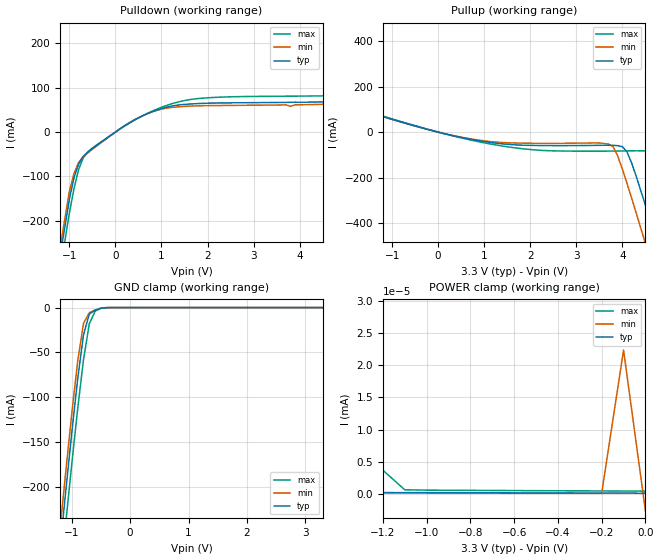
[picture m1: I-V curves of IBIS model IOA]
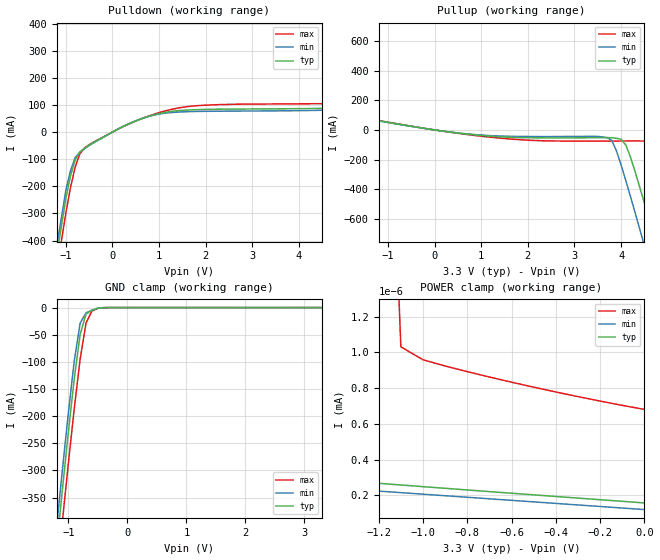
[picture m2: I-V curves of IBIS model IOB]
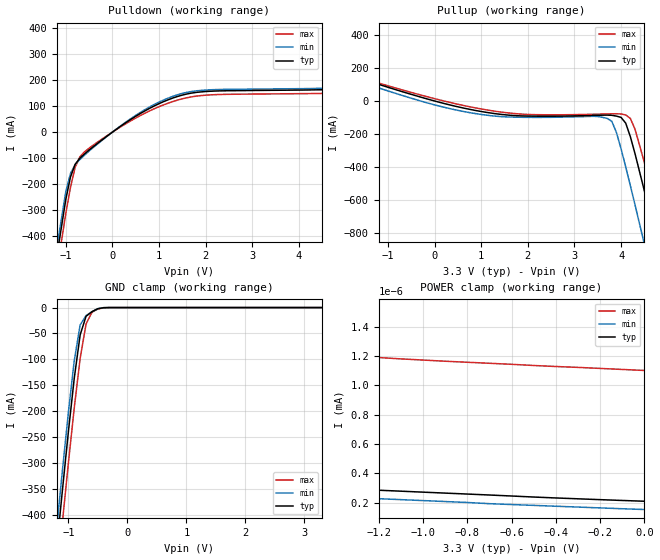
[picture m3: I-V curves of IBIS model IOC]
| IBIS file Qspan.ibs created by s2ibis2 version 2.1
[IBIS ver]   2.1
[File name]   qspn25a.ibs
[File Rev]   1.1
[Date]   10-17-2000
[Notes]   The data is simulation based
|   History : #3591862.MI003.01 - Original Model
|   #3591862.MI003.02 - Revised Power Pins.
|   #3591862.MI003.03 - Fixed IOA, IOB, and IOE Clamp
|   Characteristics and removed INE.
|   #3591862.MI003.04 - Updated with IDT formatting.
|   This is the Qspan II (CA91L862A-XXL, 17mm PBGA) IBIS
|   MODEL for a 5 V PCI signalling environment.
[Disclaimer] This model is subject to change.
   Integrated Device Technology, Inc. ("IDT") hereby grants the
   user of this IBIS model a non-exclusive, nontransferable
   license to use this IBIS model under the following terms. The
   user is granted this license only to use the IBIS model and is
   not granted rights to sell, copy (except as needed to run the
   IBIS model), rent, lease or sub-license the IBIS model in
   whole or in part, or in modified form to anyone. The User may
   modify the IBIS model to suit its specific applications, but
   rights to derivative works and such modifications shall belong
   to IDT. This IBIS model is provided on an AS IS" basis and IDT
   makes absolutely no warranty with respect to the information
   contained herein. IDT DISCLAIMS AND CUSTOMER WAIVES ALL
   WARRANTIES, EXPRESS AND IMPLIED, INCLUDING WARRANTIES OF
   MERCHANTABILITY AND FITNESS FOR A PARTICULAR PURPOSE. THE
   ENTIRE RISK AS TO QUALITY AND PERFORMANCE IS WITH THE USER
   ACCORDINGLY, IN NO EVENT SHALL IDT BE LIABLE FOR ANY DIRECT OR
   INDIRECT DAMAGES, WHETHER IN CONTRACT OR TORT, INCLUDING ANY
   LOST PROFITS OR OTHER INCIDENTAL, CONSEQUENTIAL, EXEMPLARY, OR
   PUNITIVE DAMAGES ARISING OUT OF THE USE OR APPLICATION OF THE
   IBIS model. Further, IDT reserves the right to make changes
   without notice to any product herein to improve reliability,
   function, or design. IDT does not convey any license under
   patent rights or any other intellectual property rights,
   including those of third parties. IDT is not obligated to
   provide maintenance or support for the licensed IBIS model.
[Copyright]   Copyright 2009, Integrated Device Technology, Inc. all
   rights reserved.
|   Component QSPAN
[Component]   QSPAN
[Manufacturer]   Integrated Device Technology, Inc.
[Package]
| variable   typ   min   max
R_pkg   45m   22m   75m
L_pkg   2.5nH   1.1nH   4.3nH
C_pkg   1.3pF   1.2pF   1.4pF
[Pin]  signal_name   model_name
B3	D26		IOA
C3	D27		IOA
B1	D28		IOA
D3	D29		IOA
D2	D30		IOA
C2	D31		IOA
C1	A26		IOA
E3	A27		IOA
E4	A28		IOA
E1	A29		IOA
F3	A30		IOA
F2	A31		IOA
D1	R/W		IOA
F1	DSACK1/TA	IOB
G3	DSACK0   IOB
F4	SIZ1		IOA
G2	SIZ0		IOA
G1	SDA		IOB
H3	SCL		OUTA
H4	IMSEL		INA
K8	VSS		GND
H1	TMODE1	IOD
J3	TMODE0	IOD
J4	RESETI	INB
K1	RESETO	IOF
L4	BURST/TIP	IOA
K2	TS		IOB
L2	BB/BGACK	IOB
L1	BR		OUTA
M4   REQ   IOC
N2	AD31		IOC
P1	AD30		IOC
P2	AD29		IOC
N4	AD28		IOC
N3	AD27		IOC
M1	HALT/RETRY IOB
M3	GNT		IOC
M2	RST		INC
P8	PCLK		INC
J14	BM_EN		IOD
P3	AD26		IOC
R3	AD25		IOC
R2	AD24		IOC
T2	C/BE3		IOC
T1	AD23		IOC
N5	AD22		IOC
P5	AD21		IOC
N6	AD20		IOC
R6	AD19		IOC
T5	AD18		IOC
T6	AD17		IOC
P6	AD16		IOC
N7	C/BE2		IOC
P7	FRAME		IOC
R7	IRDY		IOC
N8	TRDY		IOC
R8	DEVSEL	IOC
T7	STOP		IOC
N9	PERR		IOC
N10	PAR		IOC
R9	C/BE1		IOC
P9	AD15		IOC
T8	AD14		IOC
T9	AD13		IOC
R10	AD12		IOC
P10	AD11		IOC
N11	AD10		IOC
P11	AD9		IOC
T10	AD8		IOC
R11	C/BE0		IOC
N12	IDSEL		INC
P12	AD7		IOC
P14	AD6		IOC
T13	AD5		IOC
T14	AD4		IOC
P15	AD3		IOC
T16	AD2		IOC
N14	AD1		IOC
N15	AD0		IOC
M13	CSREG		INA
P16	CSPCI		INA
N16	TC0		IOA
L14	TC1		IOA
M16	TC2		IOA
L13	TC3		IOA
L15	BERR/TEA	IOB
L16	AS		IOB
K14	BDIP		IOA
K16	BG		INA
H15	ENID		IOD
J13	DACK/SDACK	INB
J15	DONE		INA
H16	QINT		IOE
G13	DREQ		OUTA
M14	INT		IOC
M15	SERR		IOC
G14	A0		IOA
G16	A1		IOA
G15	A2		IOA
F14	A3		IOA
F16	A4		IOA
E16	A5		IOA
F15	D0		IOA
E15	D1		IOA
E14	D2		IOA
D16	D3		IOA
D15	D4		IOA
F13	D5		IOA
F6	VSS		GND
D8	QCLK		INA
F7	VSS		GND
F8	VSS		GND
E13	D6		IOA
D14	D7		IOA
C16	D8		IOA
C15	D9		IOA
B14	D10		IOA
B15	D11		IOA
C13	A6		IOA
B16	A7		IOA
C14	A8		IOA
A15	A9		IOA
D12	A10		IOA
C11	A11		IOA
D11	A12		IOA
A13	A13		IOA
A12	A14		IOA
B11	A15		IOA
C10	DS		OUTA
D10	D12		IOA
A11	D13		IOA
D9	D14		IOA
B10	D15		IOA
C9	D16		IOA
A10	D17		IOA
B9	D18		IOA
C8	D19		IOA
A9	A16		IOA
D7	A17		IOA
B8	A18		IOA
C7	A19		IOA
A8	A20		IOA
A7	A21		IOA
B7	A22		IOA
D6	A23		IOA
C6	A24		IOA
A6	A25		IOA
B6	D20		IOA
D5	D21		IOA
A4	D22		IOA
A3	D23		IOA
B4	D24		IOA
A2	D25		IOA
H13  TCK   INF
K15  TDI   INF
K13  TDO   OUTA
J16  TMS   INF
H14  TRST   INF
G4   ENUM   IOF
K4   HS_HEALTHY IOD
H2   HS_LED   IOF
J2   HS_SWITCH  IOD
K3   PCI_DIS   IOD
J1   PME   IOF
D4   DP3   IOA
B5   DP2   IOA
C5   DP1   IOA
A5   DP0   IOA
C4   PCI_ARB_EN  IOD
B12  BIDIR_CTRL/Test1 ING
A14  RAM_WE/Test2 IOD
C12  TMODE[2]/Test3 IOD
R1	EXT_GNT[1]  OUTB
R4	EXT_GNT[2]  OUTB
T3	EXT_GNT[3]  OUTB
P4	EXT_GNT[4]  OUTB
R5	EXT_GNT[5]  OUTB
T4	EXT_GNT[6]  OUTB
T11	EXT_REQ[1]  IOC
R12	EXT_REQ[2]  IOC
N13	EXT_REQ[3]  IOC
P13	EXT_REQ[4]  IOC
T12	EXT_REQ[5]  IOC
R13	EXT_REQ[6]	  IOC
N1   VH   POWER
R15   VH   POWER
B2   VH   POWER
A16   VH   POWER
F9   VSS   GND
F10   VSS   GND
E5   VDD   POWER
F11   VSS   GND
E6   VDD   POWER
G6   VSS   GND
E7   VDD   POWER
G7   VSS   GND
G8   VSS   GND
E8   VDD   POWER
E9   VDD   POWER
E10   VDD   POWER
G9   VSS   GND
G10   VSS   GND
E11   VDD   POWER
E12   VDD   POWER
G11   VSS   GND
F5   VDD   POWER
F12   VDD   POWER
H6   VSS   GND
G5   VDD   POWER
G12   VDD   POWER
H5   VDD   POWER
H12   VDD   POWER
J5   VDD   POWER
J12   VDD   POWER
K5   VDD   POWER
K12   VDD   POWER
L5   VDD   POWER
L12   VDD   POWER
M5   VDD   POWER
M6   VDD   POWER
M7   VDD   POWER
M8   VDD   POWER
M9   VDD   POWER
M10   VDD   POWER
M11   VDD   POWER
M12   VDD   POWER
H7   VSS   GND
H8   VSS   GND
H9   VSS   GND
H10   VSS   GND
H11   VSS   GND
J6   VSS   GND
J7   VSS   GND
J8   VSS   GND
J9   VSS   GND
J10   VSS   GND
J11   VSS   GND
K6   VSS   GND
K7   VSS   GND
K9   VSS   GND
K10   VSS   GND
K11   VSS   GND
L6   VSS   GND
L7   VSS   GND
L8   VSS   GND
L9   VSS   GND
L10   VSS   GND
L11   VSS   GND
| Models and submodels in the file (14): IOA (I/O), IOB (I/O), IOC (I/O), IOD (I/O), IOE (I/O), IOF (I/O), INA (Input), INB (Input), INC (Input), IND (Input), INF (Input), ING (Input), OUTA (Output), OUTB (Output)
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|   Model IOA
[Model]   IOA
Model_type   I/O
Polarity   Non-Inverting
Vinl =   0.8000V
Vinh =   2.0000V
C_comp   5.00pF   5.00pF   5.00pF
[Voltage Range]   3.3000V   3.0000V   4.0000V
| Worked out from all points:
|   slope of the pulldown table from 0 to 0.495 V, typ, clamps not added: 15.7 ohm
|   slope of the pullup table from 0 to 0.495 V, typ, clamps not added: 21.3 ohm
|   GND clamp passes 1 mA (typ) near -0.51 V on its own axis
|   POWER clamp passes 1 mA (typ) near -2.40 V on its own axis
[Pulldown]
| voltage   I(typ)   I(min)   I(max)
-3.3V     -1.71A     -1.69A     -1.742A
-1.5V     -470.3mA   -448.8mA   -505mA
-1V       -150.9mA   -133.4mA   -182.4mA
-900mV    -103mA     -93.58mA   -127.2mA
-700mV    -54.65mA   -55.57mA   -58.25mA
200mV     14.09mA    14.63mA    13.68mA
800mV     45.98mA    45.66mA    47.26mA
1.8V      64.27mA    59.15mA    75.6mA
5.7V      75.97mA    71.08mA    91.9mA
5.9V      123.9mA    106.3mA    157.2mA
6.1V      215.3mA    196.5mA    249.6mA
6.6V      467.9mA    450mA      500.3mA
[Pullup]
| voltage   I(typ)   I(min)   I(max)
-3.3V     387.6mA    243.7mA    756.6mA
-2.9V     213mA      178.3mA    556.2mA
-2.7V     176.5mA    160.4mA    457.2mA
-2.1V     123.6mA    123.4mA    178.4mA
-1.7V     98.77mA    98.55mA    102.7mA
1.1V      -44.61mA   -40.7mA    -51.09mA
3.7V      -57.69mA   -52.46mA   -83.57mA
4.1V      -86.97mA   -225.7mA   -82.76mA
4.5V      -322.2mA   -490.2mA   -82.56mA
4.7V      -454.7mA   -625.9mA   -98.97mA
5.3V      -862.2mA   -1.037A    -447.5mA
6.6V      -1.761A    -1.94A     -1.333A
[GND_clamp]
| voltage   I(typ)   I(min)   I(max)
-3.3V     -1.709A    -1.689A    -1.741A
-1.2V     -267mA     -245.1mA   -302.2mA
-1.1V     -202mA     -180.2mA   -237.2mA
-1V       -138.9mA   -117.5mA   -173.7mA
-900mV    -79.66mA   -59.95mA   -112.9mA
-800mV    -30.51mA   -17.62mA   -58.03mA
-700mV    -7.178mA   -5.625mA   -17.92mA
-600mV    -2.869mA   -2.791mA   -3.925mA
-500mV    -689.1uA   -576.4uA   -907.2uA
-400mV    -60.78uA   -33.46uA   -124.4uA
3.3V      123.6pA    115.2pA    -80.39nA
[POWER_clamp]
| voltage   I(typ)   I(min)   I(max)
-3.3V     379.3mA    216.4mA    753.8mA
-2.5V     12.57mA    183.7nA    353mA
-2.3V     34.41uA    324.6pA    254.9mA
-2.1V     50.74nA    252.4pA    159.1mA
-2V       2.228nA    243.7pA    112.7mA
-1.9V     306pA      236pA      68.88mA
-1.3V     224.1pA    190.3pA    57.2nA
-1.2V     216.2pA    182.8pA    3.693nA
-1.1V     208.4pA    175.2pA    650.3pA
-200mV    138.8pA    107.8pA    470.3pA
-100mV    131.2pA    22.36nA    456.6pA
0V        123.7pA    -2.644nA   443.3pA
[Ramp]
| variable   typ   min   max
dV/dt_r   1.3260/0.6515n   1.1772/0.6916n   1.6662/0.5732n
dV/dt_f   1.4587/0.4496n   1.3376/0.4248n   1.7580/0.4730n
R_load = 50.0000
| End [Model] IOA
|   Model IOB
[Model]   IOB
Model_type   I/O
Polarity   Non-Inverting
Vinl =   0.8000V
Vinh =   2.0000V
C_comp   5.00pF   5.00pF   5.00pF
[Voltage Range]   3.3000V   3.0000V   4.0000V
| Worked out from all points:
|   slope of the pulldown table from 0 to 0.495 V, typ, clamps not added: 12.2 ohm
|   slope of the pullup table from 0 to 0.495 V, typ, clamps not added: 23.7 ohm
|   GND clamp passes 1 mA (typ) near -0.48 V on its own axis
|   POWER clamp passes 1 mA (typ) near -2.40 V on its own axis
[Pulldown]
| voltage   I(typ)   I(min)   I(max)
-3.3V     -2.838A    -2.805A    -2.892A
-1.5V     -779.2mA   -743.4mA   -836.9mA
-1V       -245.2mA   -214.8mA   -298.6mA
-800mV    -103.1mA   -93.75mA   -129mA
-700mV    -72.79mA   -73.87mA   -80.2mA
-400mV    -37.93mA   -39.43mA   -36.6mA
700mV     53.66mA    53.76mA    54.56mA
1.8V      82.63mA    76.05mA    97.21mA
5.7V      97.41mA    91.34mA    116.2mA
5.9V      142.3mA    124.7mA    176.8mA
6.1V      227.1mA    208.4mA    262.5mA
6.6V      462.1mA    444.4mA    495.3mA
[Pullup]
| voltage   I(typ)   I(min)   I(max)
-3.3V     355.7mA    223.3mA    694.5mA
-2.7V     160.5mA    144.4mA    419.7mA
-2.1V     111.3mA    111mA      163.4mA
-1.7V     88.9mA     88.7mA     92.54mA
1.1V      -40.15mA   -36.63mA   -45.98mA
3.7V      -51.97mA   -51.81mA   -75.23mA
3.9V      -56.38mA   -140.2mA   -74.92mA
4.1V      -100.4mA   -339.5mA   -74.5mA
4.5V      -492.3mA   -779.5mA   -75.03mA
4.7V      -712.8mA   -1.005A    -101.3mA
5.3V      -1.39A     -1.689A    -682.2mA
6.6V      -2.884A    -3.189A    -2.154A
[GND_clamp]
| voltage   I(typ)   I(min)   I(max)
-3.3V     -2.837A    -2.804A    -2.891A
-1.2V     -442.6mA   -406.3mA   -501.1mA
-1.1V     -334.7mA   -298.4mA   -393mA
-1V       -229.8mA   -194.3mA   -287.4mA
-900mV    -131.2mA   -98.64mA   -186.3mA
-800mV    -49.54mA   -28.65mA   -94.94mA
-700mV    -11.74mA   -9.656mA   -28.35mA
-600mV    -5.026mA   -4.929mA   -6.375mA
-500mV    -1.179mA   -986.4uA   -1.524mA
-400mV    -102uA     -56.15uA   -207.2uA
3.3V      157.6pA    146.2pA    27.32uA
[POWER_clamp]
| voltage   I(typ)   I(min)   I(max)
-3.3V     348.2mA    198.7mA    691.9mA
-2.4V     749.3uA    5.663nA    278.9mA
-2.3V     35.28uA    377.9pA    234mA
-2.2V     1.418uA    320.7pA    189.7mA
-2V       2.362nA    293.3pA    103.5mA
-1.9V     368.8pA    284.5pA    63.28mA
-1.7V     315.4pA    267.1pA    5.004mA
-1.2V     267.3pA    223.7pA    4.192nA
-1.1V     258pA      215.1pA    1.031nA
-1V       248.6pA    206.5pA    958.6pA
-500mV    202.7pA    163.4pA    805.2pA
0V        157.6pA    120.4pA    680.7pA
[Ramp]
| variable   typ   min   max
dV/dt_r   1.2666/0.6498n   1.1190/0.7032n   1.6008/0.5694n
dV/dt_f   1.5728/0.3692n   1.4406/0.3728n   1.8954/0.3942n
R_load = 50.0000
| End [Model] IOB
|   Model IOC
[Model]   IOC
Model_type   I/O
Polarity   Non-Inverting
Vinl =   0.8000V
Vinh =   2.0000V
C_comp   5.0000pF   5.0000pF   5.0000pF
[Temperature Range]   27.0000   0.000   70.0000
[Voltage Range]   3.3000V   3.0000V   2.8000V
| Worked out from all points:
|   slope of the pulldown table from 0 to 0.495 V, typ, clamps not added: 8.19 ohm
|   slope of the pullup table from 0 to 0.495 V, typ, clamps not added: 14.1 ohm
|   GND clamp passes 1 mA (typ) near -0.44 V on its own axis
|   POWER clamp passes 1 mA (typ) near -2.41 V on its own axis
[Pulldown]
| voltage   I(typ)   I(min)   I(max)
-3.3V     -3.036A    -3.001A    -3.093A
-1.5V     -828mA     -790.5mA   -888.3mA
-1V       -258.7mA   -228.6mA   -312.5mA
-900mV    -172.7mA   -159.4mA   -212.8mA
-800mV    -124.3mA   -125.1mA   -135.6mA
-600mV    -84.45mA   -89.19mA   -76.32mA
400mV     49.72mA    52.76mA    44.24mA
1.3V      131.7mA    138.2mA    118.1mA
5.7V      175.9mA    182.1mA    163.3mA
5.9V      218.3mA    213.7mA    220.7mA
6.1V      300mA      294.4mA    303.1mA
6.6V      528.3mA    524mA      528.9mA
[Pullup]
| voltage   I(typ)   I(min)   I(max)
-3.3V     344.3mA    275.4mA    443.3mA
-2.7V     237.3mA    218.7mA    239.5mA
-200mV    15.69mA    -8.13mA    28.9mA
1.6V      -86.11mA   -97.15mA   -73.04mA
3.7V      -85.54mA   -105.6mA   -78.4mA
3.9V      -91.57mA   -191mA     -77.35mA
4.1V      -134.7mA   -400.3mA   -84.49mA
4.3V      -320.5mA   -631.4mA   -171.9mA
4.5V      -545.8mA   -869.2mA   -373mA
4.7V      -780.9mA   -1.11A     -599.7mA
4.9V      -1.02A     -1.353A    -834.7mA
6.6V      -3.106A    -3.449A    -2.908A
[GND_clamp]
| voltage   I(typ)   I(min)   I(max)
-3.3V     -3.035A    -3A        -3.092A
-1.2V     -467.3mA   -428.9mA   -528.9mA
-1.1V     -351.9mA   -313.8mA   -413.4mA
-1V       -240.4mA   -203.1mA   -300.8mA
-900mV    -136.5mA   -102.7mA   -193.7mA
-800mV    -52.76mA   -33.54mA   -98.15mA
-700mV    -16.83mA   -15.41mA   -31.7mA
-600mV    -7.941mA   -7.925mA   -9.126mA
-500mV    -2.274mA   -1.998mA   -2.733mA
-300mV    -7.68uA    -2.34uA    -30.21uA
3.3V      210.9pA    171.2pA    1.093nA
[POWER_clamp]
| voltage   I(typ)   I(min)   I(max)
-3.3V     326.1mA    185.2mA    432.7mA
-2.5V     9.785mA    17.54nA    95.65mA
-2.4V     484.9uA    554.7pA    57.78mA
-2.3V     11.51uA    305.2pA    24.52mA
-2.1V     5.439nA    287.9pA    195.7uA
-2V       447.5pA    281.1pA    7.155uA
-1.9V     336pA      274.4pA    245.8nA
-1.7V     319.7pA    261pA      1.524nA
-1.6V     312.9pA    254.5pA    1.238nA
-1.5V     306.1pA    247.9pA    1.218nA
-1.3V     292.7pA    234.8pA    1.198nA
0V        210.9pA    154.5pA    1.102nA
[Ramp]
| variable   typ   min   max
dV/dt_r   1.5252/0.7478n   1.5510/0.6914n   1.4850/0.8731n
dV/dt_f   1.6988/0.7487n   1.7039/0.8425n   1.6714/0.7698n
R_load = 50.0000
| End [Model] IOC
